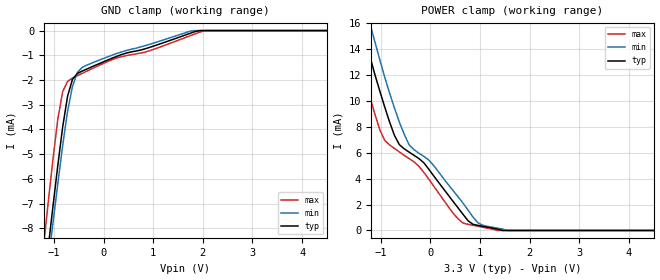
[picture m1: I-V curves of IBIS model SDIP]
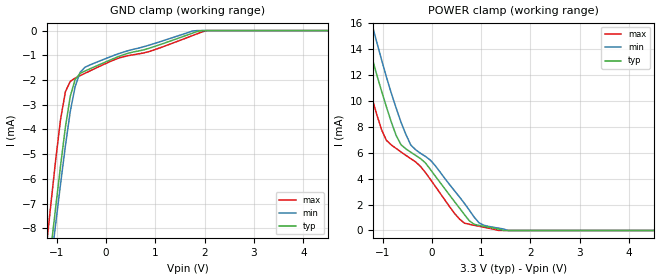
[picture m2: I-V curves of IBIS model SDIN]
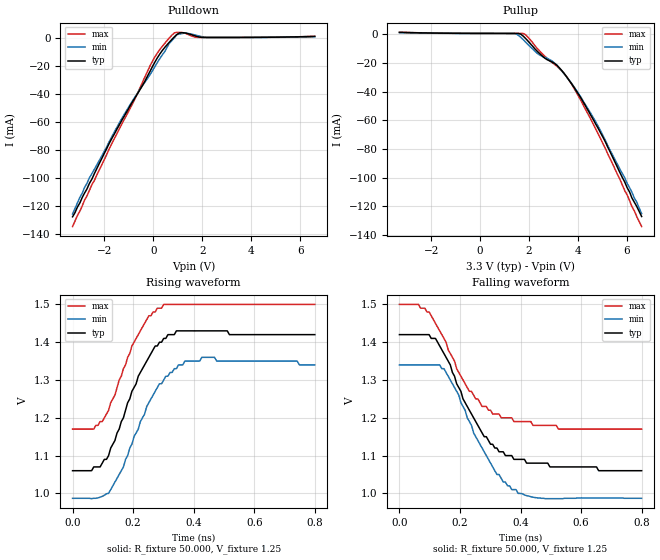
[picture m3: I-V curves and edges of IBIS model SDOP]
|   National Semiconductor Corporation
|   IBIS Model of LMH0384
[IBIS Ver]   4.2
[Comment char]  |_char
[File name]   lmh0384.ibs
[File Rev]   1.2
[Date]   09/15/2010
[Source]
[Notes]   Created by Pegah Alavi
   Revision History
   1.0  Initial Release
   1.1  Updated SDOP and SDON models
   1.2  Removed settled time from SDOP/SDON buffer tables
This model supports the SDI-Input, and SDO pins.
All of these pins are modeled with supply voltage of 3.3V
Begin IBIS Parser Results
| Do NOT edit this section manually!
Checking ...\lmh0384.ibs for IBIS 4.2 Compatibility...
WARNING - Combined Pulldown for Model: SDON Typical data is non-monotonic
WARNING - Combined Pulldown for Model: SDON Minimum data is non-monotonic
WARNING - Combined Pulldown for Model: SDON Maximum data is non-monotonic
WARNING - Combined Pulldown for Model: SDOP Typical data is non-monotonic
WARNING - Combined Pulldown for Model: SDOP Minimum data is non-monotonic
WARNING - Combined Pulldown for Model: SDOP Maximum data is non-monotonic
Errors  : 0
Warnings: 6
File Passed
[Disclaimer]
(C) Copyright National Semiconductor Corporation 2010
   All rights reserved
   National Semiconductor Corporation hereby grants
the user of this IBIS model a non-exclusive, nontransferable
license to use this IBIS model under the following terms.
Before using this IBIS model, the user should read this
license.  If the user does not accept these terms,  the
IBIS model should be returned to National within 30 days.
   The user is granted this license only to use the
IBIS model and is not granted rights to sell, load, rent,
lease or license the IBIS model in whole or in part, or in
modified form to anyone other than user. User may modify
the IBIS model to suit its specific applications but rights
to derivative works and such modifications shall belong to
National.
   This IBIS model is provided on an "AS IS" basis and
National makes absolutely no warranty with respect to the
information contained herein.NATIONAL DISCLAIMS AND CUSTOMER
WAIVES ALL WARRANTIES, EXPRESS OR IMPLIED, INCLUDING
WARRANTIES OF MERCHANTABILITY OR FITNESS FOR A PARTICULAR
PURPOSE. The entire risk as to quality and performance is
with the Customer. ACCORDINGLY, IN NO EVENT SHALL THE
COMPANY BE LIABLE FOR ANY DAMAGES, WHETHER IN CONTRACT OR
TORT,INCLUDING ANY LOST PROFITS OR OTHER INCIDENTAL,
CONSEQUENTIAL, EXEMPLARY, OR PUNITIVE DAMAGES ARISING OUT
OF THE USE OR APPLICATION OF THE IBIS model provided in
this package.Further, National reserves the right to make
changes without notice to any product herein to improve
reliability, function, or design. National does not convey
any license under patent rights or any other intellectual
property rights, including those of third parties.
   National is not obligated to provide maintenance or support
for the licensed IBIS model.
[Component]   LMH0384
[Manufacturer]  National Semiconductor
[Package]
|   typ   min   max
R_pkg   207e-03   207e-03   207e-03
L_pkg   7.63e-10   7.63e-10   7.63e-10
C_pkg   1.92e-13   1.92e-13   1.92e-13
[PIN]   signal_name   model_name   R_pin   L_pin   C_pin
1   Vee   GND
2   SDI   SDIP   0.263   8.51e-10   1.80e-13
3   SDIb   SDIN   0.265   8.63e-10   1.80e-13
4   SPI_EN   NC
5   AEC+   NC
6   AEC-   NC
7   BYPASS   NC
8   MuteREF   NC
9   Vee   GND
10   SDOb   SDON   0.150   6.64e-10   2.06e-13
11   SDO   SDOP   0.152   6.74e-10   2.03e-13
12   AUTO_SLEEP   NC
13   Vcc   POWER
14   MUTE   NC
15   CDb   NC
16   Vcc   POWER
[Diff_pin]   inv_pin   vdiff   tdelay_typ   tdelay_min   tdelay_max
| The '+' pin is Diff_pin and the '-' pin is the inv_pin
2   3   0.050   0 0 0
11   10   0.000   0 0 0
| Models and submodels in the file (4): SDIP (Input), SDIN (Input), SDOP (Output), SDON (Output)
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|   Model SDIP
[Model]   SDIP
Model_type   Input
Polarity   Non-Inverting
Vinl=0.8V
Vinh=2.0V
C_comp   500fF   480fF   520fF
[Temperature Range]   25.0   85.0   -40.0
[Voltage Range]   3.300V   3.135V   3.465V
[GND Clamp]
|Voltage   I(typ)   I(min)   I(max)
-3.399V   -53.67mA   -52.93mA   -53.54mA
-1.221V   -10.64mA   -11.17mA   -8.938mA
-1.122V   -8.892mA   -9.492mA   -7.072mA
-1.023V   -7.168mA   -7.84mA    -5.255mA
-924mV    -5.487mA   -6.223mA   -3.607mA
-825mV    -3.913mA   -4.669mA   -2.476mA
-726mV    -2.66mA    -3.271mA   -2.056mA
-627mV    -1.977mA   -2.265mA   -1.923mA
-528mV    -1.735mA   -1.694mA   -1.825mA
-132mV    -1.376mA   -1.231mA   -1.447mA
2.046V    0A         0A         0A
6.798V    0A         0A         0A
[Power Clamp]
|Voltage   I(typ)   I(min)   I(max)
-3.399V   97.59mA    109.5mA    86.47mA
-1.617V   19.58mA    24.39mA    16.35mA
-1.419V   16.45mA    19.33mA    13.16mA
-1.221V   13.46mA    16.03mA    10.34mA
-924mV    9.577mA    11.89mA    6.977mA
-627mV    6.634mA    8.376mA    6.072mA
-429mV    6.055mA    6.614mA    5.552mA
-132mV    5.227mA    5.731mA    4.484mA
660mV     1.231mA    2.096mA    566.7uA
957mV     391.4uA    588.8uA    326.6uA
1.551V    0A         0A         0A
6.798V    0A         0A         0A
|   Model SDIN
[Model]   SDIN
Model_type   Input
Polarity   Inverting
Vinl=0.8V
Vinh=2.0V
C_comp   500fF   480fF   520fF
[Temperature Range]   25.0   85.0   -40.0
[Voltage Range]   3.300V   3.135V   3.465V
[GND Clamp]
|Voltage   I(typ)   I(min)   I(max)
-3.399V   -53.67mA   -52.93mA   -53.54mA
-1.221V   -10.64mA   -11.17mA   -8.938mA
-1.122V   -8.892mA   -9.492mA   -7.072mA
-1.023V   -7.168mA   -7.84mA    -5.255mA
-924mV    -5.487mA   -6.223mA   -3.607mA
-825mV    -3.913mA   -4.669mA   -2.476mA
-726mV    -2.66mA    -3.271mA   -2.056mA
-627mV    -1.977mA   -2.265mA   -1.923mA
-528mV    -1.735mA   -1.694mA   -1.825mA
-132mV    -1.376mA   -1.231mA   -1.447mA
2.046V    0A         0A         0A
6.798V    0A         0A         0A
[Power Clamp]
|Voltage   I(typ)   I(min)   I(max)
-3.399V   97.59mA    109.5mA    86.47mA
-1.617V   19.58mA    24.39mA    16.35mA
-1.419V   16.45mA    19.33mA    13.16mA
-1.221V   13.46mA    16.03mA    10.34mA
-924mV    9.577mA    11.89mA    6.977mA
-627mV    6.634mA    8.376mA    6.072mA
-429mV    6.055mA    6.614mA    5.552mA
-132mV    5.227mA    5.731mA    4.484mA
660mV     1.231mA    2.096mA    566.7uA
957mV     391.4uA    588.8uA    326.6uA
1.551V    0A         0A         0A
6.798V    0A         0A         0A
|   Model SDOP
[Model]  SDOP
Model_type Output
Polarity   Non-Inverting
Vmeas =  1.2V
Rref =   50.0000
Vref =   1.20V
C_comp   542.2fF   513.0fF   577.4fF
[Temperature Range]   34.0000   94.0000   -31.0000
[Voltage Range]   3.3000V   3.1350V   3.4650V
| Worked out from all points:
|   slope of the pulldown table from 0 to 0.495 V, typ, clamps not added: 37.7 ohm
|   slope of the pullup table from 0 to 0.495 V, typ, clamps not added: 38.1 kohm
|   rising waveform, R_fixture 50.000, V_fixture 1.25: 20-80 % time 109ps typ, 113ps min, 102ps max; typ from 1.06 V to 1.42 V
|   falling waveform, R_fixture 50.000, V_fixture 1.25: 20-80 % time 137ps typ, 127ps min, 139ps max; typ from 1.42 V to 1.06 V
[Pulldown]
|Voltage   I(typ)   I(min)   I(max)
-3.3V     -128mA     -126mA     -135mA
-2.61V    -104mA     -100mA     -109mA
-1.32V    -59.9mA    -58.5mA    -62.7mA
-825mV    -44.9mA    -44.2mA    -46.2mA
-33mV     -20.3mA    -23.3mA    -16.4mA
363mV     -8.95mA    -12.1mA    -5.95mA
660mV     -2.8mA     -3.59mA    273uA
858mV     928uA      193uA      3.75mA
1.06V     3.72mA     2.99mA     4.23mA
1.35V     3.58mA     3.59mA     3.19mA
2.05V     540uA      862uA      551uA
6.6V      1.31mA     993uA      1.3mA
[Pullup]
|Voltage   I(typ)   I(min)   I(max)
-3.3V     1.31mA     993uA      1.3mA
1.35V     516uA      476uA      550uA
1.65V     98.8uA     -2.04mA    546uA
1.85V     -2.87mA    -5.37mA    -326uA
2.34V     -12mA      -13.4mA    -10.1mA
2.64V     -16.7mA    -16.2mA    -15.3mA
3.14V     -21.7mA    -21.7mA    -22.4mA
3.53V     -29.6mA    -29.7mA    -29.5mA
3.93V     -39.5mA    -39mA      -40.5mA
4.92V     -68.7mA    -67.3mA    -72.8mA
5.91V     -103mA     -100mA     -109mA
6.6V      -127mA     -125mA     -134mA
[Ramp]
|variable   typ   min   max
dV/dt_r   215.21m/105.7p   214.09m/131.1p   200.36m/99.93p
dV/dt_f   215.31m/126.8p   213.97m/129.6p   200.43m/123.8p
R_load  = 50
[Rising Waveform]
R_fixture = 50.000
V_fixture = 1.25
V_fixture_min = 1.125
V_fixture_max = 1.375
|  time   V(typ)   V(min)   V(max)
0s        1.06V      987mV      1.17V
70ps      1.07V      987mV      1.17V
119ps     1.1V       1V         1.22V
168ps     1.2V       1.07V      1.33V
217ps     1.31V      1.17V      1.42V
252ps     1.36V      1.24V      1.47V
315ps     1.42V      1.31V      1.5V
371ps     1.43V      1.35V      1.5V
427ps     1.43V      1.36V      1.5V
800ps     1.42V      1.34V      1.5V
[Falling Waveform]
R_fixture = 50.000
V_fixture = 1.25
V_fixture_min = 1.125
V_fixture_max = 1.375
|  time   V(typ)   V(min)   V(max)
0s        1.42V      1.34V      1.5V
84ps      1.42V      1.34V      1.49V
119ps     1.41V      1.34V      1.45V
147ps     1.37V      1.33V      1.41V
231ps     1.22V      1.19V      1.27V
280ps     1.15V      1.11V      1.23V
322ps     1.12V      1.05V      1.21V
392ps     1.09V      1V         1.19V
525ps     1.07V      986mV      1.17V
800ps     1.06V      987mV      1.17V
